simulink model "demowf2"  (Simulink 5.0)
settings: Solver=ode4  StartTime=0.0  StopTime=100  FixedStep=0.1  RelTol=1e-3
libraries: simulink_extras x5, simulink x3, MarineGNC x2

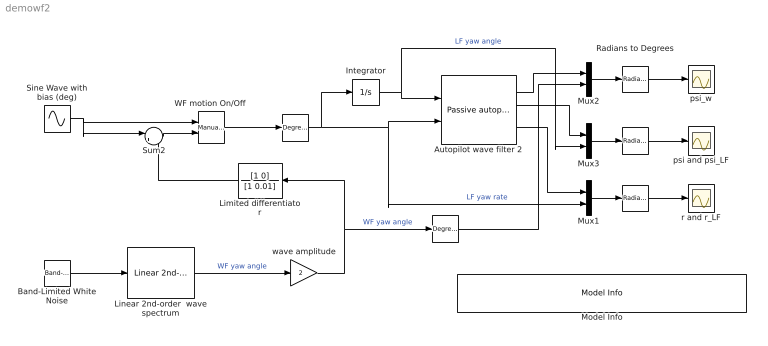
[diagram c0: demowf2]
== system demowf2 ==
  " " : simulink_extras/Transformations/Radians to Degrees
  "  " : simulink_extras/Transformations/Radians to Degrees
  "   " : simulink_extras/Transformations/Degrees to Radians
  "        " : simulink_extras/Transformations/Degrees to Radians
  Autopilot wave filter 2 : MarineGNC/Navigation/Wave filters/Passive autopilot wave filter 2  lambda=0.1  w_o=1.2  K4=0  zeta_n=0.01  w_c=2  T_b=100
  Band-Limited White Noise : simulink/Sources/Band-Limited White Noise  Cov=[1]  Ts=0.1  seed=[23341]
  Integrator : Integrator
  Limited differentiator : TransferFcn  Orientation=left  Numerator=[1 0]  Denominator=[1 0.01]
  Linear 2nd-order  wave spectrum : MarineGNC/Models/Waves, wind and currents/Linear 2nd-order  wave spectrum  sigma=0.5  w_0=1.2  lambda=0.1
  Model Info : simulink/Model-Wide Utilities/Model Info  InitialBlockCM=None  BlockCM=None  Frame=on  DisplayStringWithTags=|  HorizontalTextAlignment=Left  LeftAlignmentValue=0.02  SourceBlockDiagram=demowf2  TagMaxNumber=20
      | Wave filter demo using compass and gyro measurements
      | %<Creator>Author: Thor I. Fossen
      | %<LastModificationDate>
  Mux1 : Mux  Inputs=2
  Mux2 : Mux  Inputs=2
  Mux3 : Mux  Inputs=2
  "Radians to Degrees  " : simulink_extras/Transformations/Radians to Degrees
  Sine Wave with bias (deg) : Sin  Amplitude=0.5  Frequency=0.1  SampleTime=0
  Sum2 : Sum  Inputs=|++
  "WF motion On/Off " : simulink/Signal Routing/Manual Switch  sw=0  action=0
  psi and psi_LF : Scope
  psi_w : Scope
  r and r_LF : Scope
  wave amplitude : Gain  Gain=2
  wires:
  Band-Limited White Noise/1 -> Linear 2nd-order  wave spectrum/1
  Mux2/1 -> "Radians to Degrees  "/1
  "Radians to Degrees  "/1 -> psi_w/1
  " "/1 -> psi and psi_LF/1
  Mux1/1 -> "  "/1
  "  "/1 -> r and r_LF/1
  "WF motion On/Off "/1 -> "        "/1
  Linear 2nd-order  wave spectrum/1 -> wave amplitude/1  "WF yaw angle"
  Autopilot wave filter 2/3 -> Mux1/1
  Integrator/1 -> Mux3/2, Autopilot wave filter 2/1  "LF yaw angle"
  Sine Wave with bias (deg)/1 -> "WF motion On/Off "/1, Sum2/1
  Sum2/1 -> "WF motion On/Off "/2
  "        "/1 -> Mux1/2, Autopilot wave filter 2/2, Integrator/1  "LF yaw rate"
  Autopilot wave filter 2/2 -> Mux3/1
  Mux3/1 -> " "/1
  wave amplitude/1 -> "   "/1, Limited differentiator/1  "WF yaw angle"
  Limited differentiator/1 -> Sum2/2
  Autopilot wave filter 2/1 -> Mux2/1
  "   "/1 -> Mux2/2
